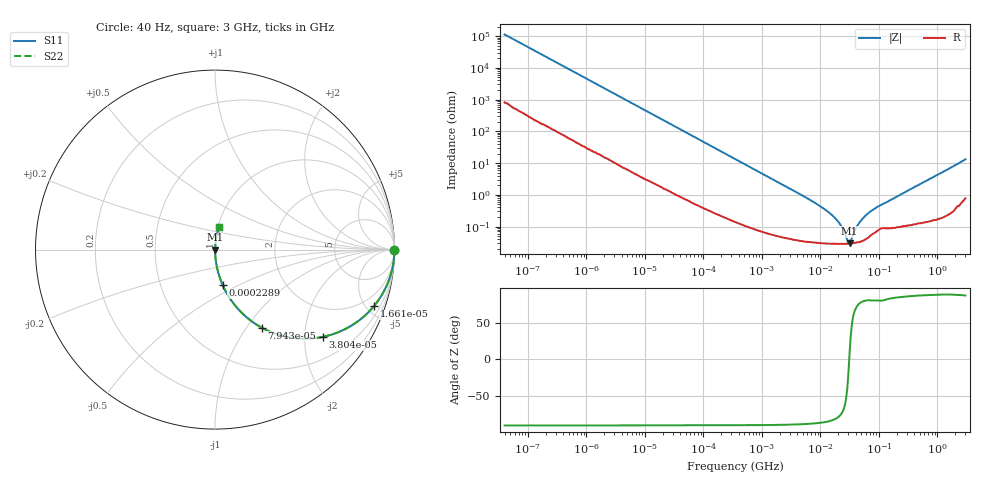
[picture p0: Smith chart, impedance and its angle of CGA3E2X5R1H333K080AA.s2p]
! S-parameter Generated by TDK Corporation
! Copyright(C) 2015 TDK Corporation.
! All Rights Reserved.
! TDK P/N: CGA3E2X5R1H333K080AA (Multilayer Ceramic Chip Capacitors)
! Property: C=33nF
! Size(LxWxT): 1.6x0.8x0.8mm, 0.063x0.031x0.031inches
! Model Type: s2p (Touchstone File Format Version 1.0)
! Frequency: DC=Yes Start=0.00004MHz Stop=3000MHz 396points Log-sweep
! Note: This model was converted from impedance.
! Model Generated on Jun. 23, 2015
! Hash(MD5):
! Port Assignments:
!  1 ---| |--- 2
! Applicable Conditions:
!  Temperature = 25 degC
!  DC Bias Voltage = 0 V
!  Small Signal Operation
! Terms and conditions regarding TDK Simulation Models
! (1)This simulation model is being provided solely for informational purposes. Please refer to the specifications of the products in terms of detailed characteristics of such products.
! (2)In no event shall TDK Corporation of any of its subsidiaries be liable for any loss or damage arising, directly or indirectly,
!  From any information contained in this simulation model, including, but not limited to loss or damages arising from any inaccuracies, omissions or errors in connection with such information.
! (3)Any and all copyrights on this simulation model are owned by TDK Corporation.
!  Duplication or redistribution of this simulation model without prior written permission from TDK Corporation is prohibited.
! (4)This simulation model is subject to any modification or change without any prior notice.
! (5)Neither TDK Corporation nor any of its subsidiaries shall make any warranty, express or implied,
!  Including but not limited to the correctness, implied warranties of merchantability and fitness for a particular purpose with respect to this simulation models.
! (6)The use of this simulation model shall be deemed to have consented to the terms and conditions hereof.
# MHz S MA R 50
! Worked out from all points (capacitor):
!   395 points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, 40 Hz to 3 GHz, reference 50 ohm
!   read as one part in series: C = 35.2 nF near 41.88 Hz
!   lowest |Z| = 29.8 mohm at 31.5 MHz (marker M1)
!   series resonance near 31.03 MHz, so ESL is about 750 pH
!   S11 on the Smith chart (normalised r, x): 40 Hz: open; 16.61 kHz: 1.04, -5.59; 38.04 kHz: 1.02, -2.45; 79.43 kHz: 1.01, -1.18; 228.9 kHz: 1.00, -0.41; 3 GHz: 1.02, +0.26
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4e-05  1 -0.1  0.0008871 89.5  0.0008871 89.5  1 -0.1
0.000834128  0.9997 -1.0  0.01818 88.6  0.01818 88.6  0.9997 -1.0
0.004794644  0.994 -5.9  0.1031 83.7  0.1031 83.7  0.994 -5.9
0.01661185  0.9395 -19.6  0.336 70.0  0.336 70.0  0.9395 -19.6
0.01739424  0.9344 -20.5  0.3499 69.1  0.3499 69.1  0.9344 -20.5
0.03803578  0.772 -39.0  0.6299 50.5  0.6299 50.5  0.772 -39.0
0.07943131  0.5057 -59.2  0.8587 30.4  0.8587 30.4  0.5057 -59.2
0.1317813  0.3345 -70.0  0.9395 19.5  0.9395 19.5  0.3345 -70.0
0.2289304  0.201 -77.9  0.9777 11.6  0.9777 11.6  0.201 -77.9
0.3464102  0.1348 -81.7  0.9895 7.7  0.9895 7.7  0.1348 -81.7
1.146211  0.04137 -86.8  0.9985 2.4  0.9985 2.4  0.04137 -86.8
7.22376  0.006305 -86.8  0.9997 0.4  0.9997 0.4  0.006305 -86.8
13.14015  0.00303 -84.3  0.9997 0.2  0.9997 0.2  0.00303 -84.3
18.98891  0.00162 -79.7  0.9997 0.1  0.9997 0.1  0.00162 -79.7
23.90217  0.0008732 -70.8  0.9997 0.0  0.9997 0.0  0.0008732 -70.8
30.08671  0.0003079 -18.3  0.9997 0.0  0.9997 0.0  0.0003079 -18.3
31.50375  0.0002981 9.3  0.9997 -0.0  0.9997 -0.0  0.0002981 9.3
41.52283  0.0009804 71.1  0.9997 -0.1  0.9997 -0.1  0.0009804 71.1
54.72828  0.001929 79.0  0.9996 -0.1  0.9996 -0.1  0.001929 79.0
86.71344  0.003802 79.9  0.9993 -0.2  0.9993 -0.2  0.003802 79.9
150.6385  0.006539 81.9  0.9991 -0.4  0.9991 -0.4  0.006539 81.9
3000  0.1291 79.2  0.984 -7.4  0.984 -7.4  0.1291 79.2
